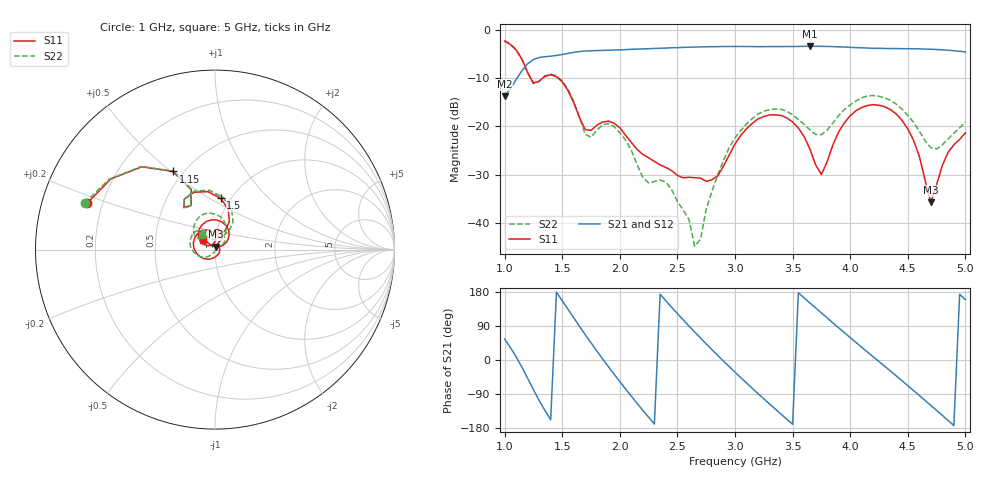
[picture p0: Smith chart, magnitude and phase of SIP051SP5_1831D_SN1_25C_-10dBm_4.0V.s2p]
# GHz  S  dB  R  50
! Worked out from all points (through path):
!   81 points, 1 GHz to 5 GHz, reference 50 ohm
!   highest |S21| = -3.47 dB at 3.65 GHz (marker M1); lowest = -13.8 dB at 1 GHz (marker M2)
!   lowest |S11| = -35.8 dB at 4.7 GHz (marker M3), VSWR 1.03, Z = 50.3 + j1.6 ohm
!   |S11| at or under -10 dB: 1.225 GHz to 1.333 GHz (108 MHz wide, 8.44 % of centre); 1.462 GHz to end of sweep
!   |S22| runs from -44.8 to -2.3 dB; largest |S21 - S12| = 0.0047
!   S11 on the Smith chart (normalised r, x): 1 GHz: 0.14, +0.17; 1.15 GHz: 0.44, +0.51; 1.5 GHz: 0.90, +0.56; 5 GHz: 0.87, +0.10
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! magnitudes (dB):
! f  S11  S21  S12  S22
! 1 GHz  -2.4  -13.8  -13.8  -2.3
! 1.15 GHz  -6.1  -8.5  -8.5  -6.1
! 1.25 GHz  -11.1  -6.2  -6.2  -11.2
! 1.5 GHz  -10.8  -5.2  -5.1  -10.6
! 1.7 GHz  -20.7  -4.4  -4.5  -21.7
! 1.95 GHz  -19.4  -4.2  -4.2  -20.1
! 2.2 GHz  -25.8  -4.0  -4.0  -30.6
! 2.35 GHz  -28.0  -3.9  -3.9  -31.1
! 2.6 GHz  -30.6  -3.7  -3.7  -39.3
! 2.65 GHz  -30.6  -3.6  -3.6  -44.8
! 2.85 GHz  -30.3  -3.5  -3.5  -30.1
! 3 GHz  -23.7  -3.5  -3.5  -22.4
! 3.35 GHz  -17.7  -3.5  -3.5  -16.4
! 3.65 GHz  -24.7  -3.5  -3.5  -20.8
! 3.7 GHz  -28.0  -3.5  -3.5  -21.7
! 3.75 GHz  -30.0  -3.5  -3.5  -21.7
! 4.05 GHz  -16.8  -3.7  -3.7  -14.8
! 4.35 GHz  -16.6  -3.9  -3.9  -14.6
! 4.55 GHz  -22.9  -4.0  -4.0  -19.2
! 4.7 GHz  -35.8  -4.1  -4.1  -24.5
! 4.85 GHz  -25.4  -4.3  -4.3  -22.6
! 5 GHz  -21.4  -4.6  -4.6  -19.1
